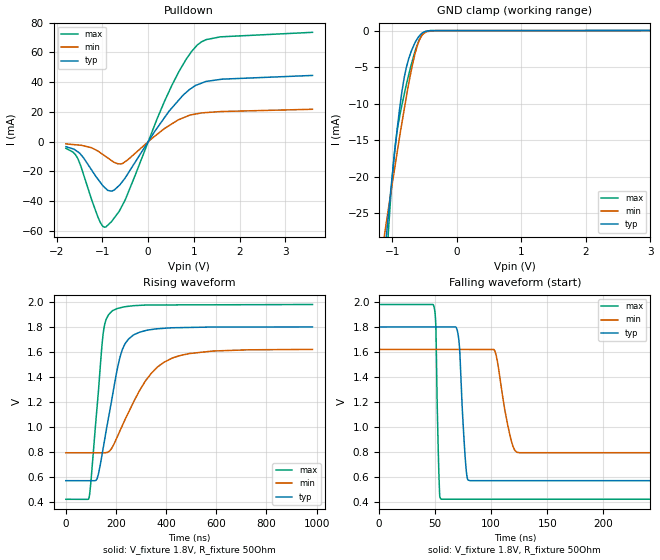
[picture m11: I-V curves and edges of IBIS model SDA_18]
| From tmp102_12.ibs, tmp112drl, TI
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|   SDA_18  1.8V digital I/O open drain Model
[Model] SDA_18
Model_type   I/O_open_drain
| Signals   SDA(6)
Polarity   Non-Inverting
Enable   Active-Low
Vinl = 0.54
Vinh = 1.26
Vmeas = 0.9
Vref = 0.9
Cref = 15pF
Rref = 50
|   typ   min   max
|   (nom PVT)   (Fast PVT)   (slow PVT)
|   output low
|C_comp   1.2319880e-10  6.9039530e-11  1.8866880e-10
| Where   nom PVT is  Nominal Process, 1.8V, 27C
|   Fast PVT is Strong Process, 1.98V, 125C
|   Slow PVT is Weak Process, 1.62V, -40C
|   output high
C_comp   1.4125270e-12  1.4056540e-12   1.4138660e-12
| Where   nom PVT is  Nominal Process, 1.5V, 27C
|   Fast PVT is Strong Process, 1.6V, -40C
|   Slow PVT is Weak Process, 1.4V, 125C
[Voltage Range]   1.8   1.62   1.98
[Temperature Range]   27   125   -40
|Ambient Temperature   27   125   -40
[Pullup Reference]   1.8   1.62   1.98
[Pulldown Reference]   0   0   0
[Power Clamp Reference]   1.8   1.62   1.98
[GND Clamp Reference]   0   0   0
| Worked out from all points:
|   slope of the pulldown table from 0 to 0.27 V, typ, clamps not added: 21.7 ohm
|   GND clamp passes 1 mA (typ) near -0.60 V on its own axis
|   falling waveform, V_fixture 1.8V, R_fixture 50Ohm: 20-80 % time 4.12ns typ, 9.34ns min, 2.06ns max; typ from 1.8 V to 0.567 V
|   rising waveform, V_fixture 1.8V, R_fixture 50Ohm: 20-80 % time 67.8ns typ, 140ns min, 37.8ns max; typ from 0.567 V to 1.8 V
[Pulldown]
|   Voltage   I(typ)   I(min)   I(max)
-1.8V     -3.345mA   -1.488mA   -4.466mA
-1.542V   -6.77mA    -2.212mA   -11.14mA
-1.097V   -25.29mA   -6.332mA   -50.83mA
-1.002V   -29.18mA   -8.379mA   -56.53mA
-927mV    -31.48mA   -9.99mA    -57.37mA
-790.3mV  -33.24mA   -12.94mA   -53.29mA
-553.7mV  -26.44mA   -14.55mA   -42.18mA
524.2mV   22.84mA    12.08mA    38.19mA
819.6mV   32.76mA    16.7mA     54.81mA
1.072V    38.22mA    18.8mA     64.88mA
1.584V    41.87mA    20.25mA    70.48mA
3.595V    44.53mA    21.79mA    73.51mA
[GND Clamp]
|   Voltage   I(typ)   I(min)   I(max)
-1.8V     -98.63mA   -69.3mA    -151.9mA
-1.123V   -31.37mA   -28.27mA   -37.25mA
-1.071V   -26.52mA   -25.22mA   -29.53mA
-1.05V    -24.55mA   -23.95mA   -26.52mA
-992.4mV  -19.45mA   -20.68mA   -19.47mA
-942.7mV  -15.24mA   -17.87mA   -15.08mA
-877.8mV  -10.3mA    -14.22mA   -11.55mA
-815.1mV  -6.58mA    -10.94mA   -8.851mA
-673.2mV  -2.225mA   -4.22mA    -3.733mA
-538mV    -356.5uA   -676.7uA   -603.7uA
-327.8mV  -14.71uA   -7.212uA   -18.83uA
3.595V    0A         0A         0A
[POWER Clamp]
|   SCR cell for ESD function. Effects occurr above VDD x 2
|   Voltage   I(typ)   I(min)   I(max)
-1.8V     0A         0A         0A
0V        0A         0A         0A
3.6V      0A         0A         0A
[Ramp]
R_load = 50
|   typ   min   max
dV/dt_r   0.739849/6.77384e-008   0.49742/1.39116e-007  0.937297/3.77456e-008
dV/dt_f   0.739849/4.11329e-009   0.49742/9.27154e-009  0.937297/2.05518e-009
[Falling Waveform]
V_fixture = 1.8V
V_fixture_min = 1.62V
V_fixture_max = 1.98V
R_fixture = 50Ohm
C_fixture = 0F
|   Time   V(typ)   V(min)   V(max)
0s        1.8V       1.62V      1.98V
48.69ns   1.8V       1.62V      1.969V
50.56ns   1.8V       1.62V      1.8V
53.93ns   1.8V       1.62V      462.8mV
55.52ns   1.8V       1.62V      418.6mV
70.51ns   1.736V     1.62V      418.5mV
80.99ns   567.5mV    1.619V     418.5mV
103.1ns   567.5mV    1.61V      418.5mV
125.7ns   567.5mV    791.6mV    418.5mV
983.5ns   566.9mV    791mV      417.8mV
[Rising Waveform]
V_fixture = 1.8V
V_fixture_min = 1.62V
V_fixture_max = 1.98V
R_fixture = 50Ohm
C_fixture = 0F
|   Time   V(typ)   V(min)   V(max)
0s        566.9mV    791mV      417.8mV
92.44ns   566.8mV    791mV      429.8mV
124.3ns   582.2mV    791mV      1.153V
148.7ns   826.5mV    791mV      1.744V
183.1ns   1.217V     828mV      1.925V
217.4ns   1.569V     974.1mV    1.954V
250.1ns   1.704V     1.116V     1.966V
341.2ns   1.779V     1.429V     1.976V
422ns     1.793V     1.548V     1.977V
983.5ns   1.8V       1.62V      1.98V
